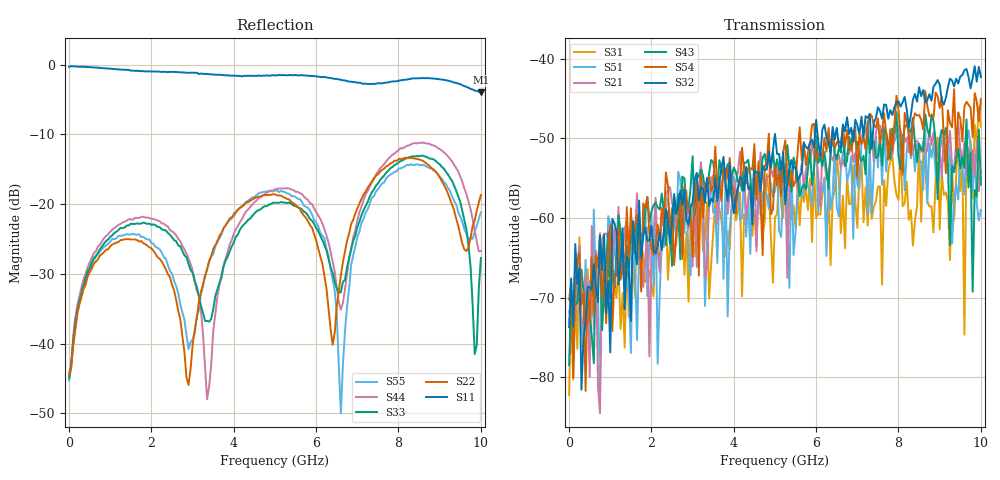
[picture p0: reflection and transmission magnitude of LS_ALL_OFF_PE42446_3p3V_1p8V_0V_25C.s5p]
!Agilent Technologies,N5230C,MY49001984,A.09.33.09
!Agilent N5230C: A.09.33.09
!Date: Tuesday, July 09, 2024 13:05:13
!Correction: S11(Full 5 Port(1,2,3,4,5))
!S12(Full 5 Port(1,2,3,4,5))
!S13(Full 5 Port(1,2,3,4,5))
!S14(Full 5 Port(1,2,3,4,5))
!S15(Full 5 Port(1,2,3,4,5))
!S21(Full 5 Port(1,2,3,4,5))
!S22(Full 5 Port(1,2,3,4,5))
!S23(Full 5 Port(1,2,3,4,5))
!S24(Full 5 Port(1,2,3,4,5))
!S25(Full 5 Port(1,2,3,4,5))
!S31(Full 5 Port(1,2,3,4,5))
!S32(Full 5 Port(1,2,3,4,5))
!S33(Full 5 Port(1,2,3,4,5))
!S34(Full 5 Port(1,2,3,4,5))
!S35(Full 5 Port(1,2,3,4,5))
!S41(Full 5 Port(1,2,3,4,5))
!S42(Full 5 Port(1,2,3,4,5))
!S43(Full 5 Port(1,2,3,4,5))
!S44(Full 5 Port(1,2,3,4,5))
!S45(Full 5 Port(1,2,3,4,5))
!S51(Full 5 Port(1,2,3,4,5))
!S52(Full 5 Port(1,2,3,4,5))
!S53(Full 5 Port(1,2,3,4,5))
!S54(Full 5 Port(1,2,3,4,5))
!S55(Full 5 Port(1,2,3,4,5))
!S5P File: Measurements: <S11,S12,S13,S14,S15>,
!<S21,S22,S23,S24,S25>,
!<S31,S32,S33,S34,S35>,
!<S41,S42,S43,S44,S45>,
!<S51,S52,S53,S54,S55>:
# Hz S  dB  R 50
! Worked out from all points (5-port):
!   201 points, 10 MHz to 10 GHz, reference 50 ohm
!   strongest paths, dB at 10 MHz, 2.507 GHz, 5.005 GHz, 7.503 GHz, 10 GHz:
!     S32: -73.7, -60.4, -49.4, -46.1, -42.3
!     S54: -70.3, -58.7, -53.6, -47.5, -45.0
!     S43: -78.5, -66.0, -54.1, -52.3, -55.8
!     S21: -72.7, -58.1, -53.1, -48.3, -54.1
!     S51: -71.7, -62.8, -56.5, -53.7, -59.0
!     S31: -82.3, -64.5, -59.9, -56.0, -48.5
!   lowest |S11| = -3.9 dB at 10 GHz (marker M1), VSWR 4.48, Z = 178 - j87.4 ohm
!   |S11| at or under -10 dB: nowhere
